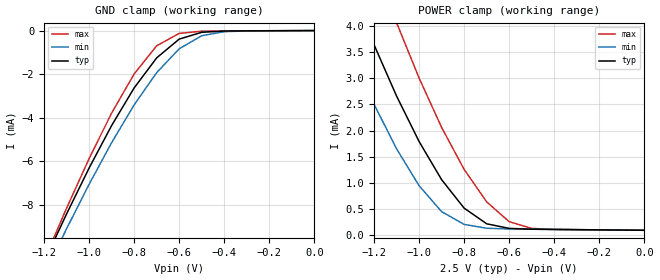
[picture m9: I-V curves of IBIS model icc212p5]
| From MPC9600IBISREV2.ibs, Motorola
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|This is a Model of a CMOS input with a 25,000 ohm Pull_down at 2.5V
[Model]   icc212p5
Model_type   Input
Vmeas=1.25
Vinl=.7
Vinh=1.7
| Variable   typ   min   max
C_comp   5p   5p   5p
[Temperature Range]   27.00   100.00   -45.00
[Power Clamp Reference]   2.50V   2.25V   2.75V
[Gnd Clamp Reference]   0.000V   0.000V   0.000V
[Voltage Range]   2.50V   2.25V   2.75V
[Pulldown Reference]   0.000V   0.000V   0.000V
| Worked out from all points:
|   GND clamp passes 1 mA (typ) near -0.67 V on its own axis
|   POWER clamp passes 1 mA (typ) near -0.89 V on its own axis
[GND_clamp]
| voltage   I(typ)   I(min)   I(max)
-2.5V     -42.42mA   -42.05mA   -44.22mA
-1.2V     -10.62mA   -11.21mA   -10.54mA
-1.1V     -8.405mA   -9.084mA   -8.143mA
-1V       -6.302mA   -7.048mA   -5.871mA
-900mV    -4.353mA   -5.139mA   -3.783mA
-800mV    -2.629mA   -3.405mA   -1.989mA
-700mV    -1.25mA    -1.928mA   -696.5uA
-600mV    -391uA     -834.6uA   -129.1uA
-500mV    -78.3uA    -235.5uA   -27.92uA
-400mV    -21.22uA   -49.71uA   -16.12uA
1.08fV    -5.997pA   -4.086nA   -2.25pA
[POWER_clamp]
| voltage   I(typ)  I(min)  I(max)
-2.5V     21.11mA    19.27mA    23.62mA
-1.4V     5.858mA    4.506mA    7.709mA
-1.3V     4.709mA    3.46mA     6.427mA
-1.2V     3.638mA    2.502mA    5.205mA
-1.1V     2.659mA    1.653mA    4.058mA
-1V       1.792mA    949.5uA    3.003mA
-900mV    1.064mA    454.7uA    2.061mA
-800mV    521.3uA    211.1uA    1.26mA
-700mV    222.9uA    137.8uA    641uA
-600mV    134.9uA    124uA      262.6uA
-500mV    119.8uA    118.9uA    134.9uA
1.08fV    99.01uA    99.01uA    99.01uA
